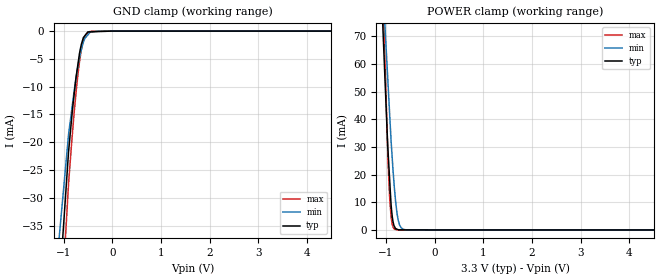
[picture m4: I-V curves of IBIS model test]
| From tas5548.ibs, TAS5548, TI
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|   test Model
[Model]   test
Model_type   Input
Vinl = 0.8
Vinh = 2
|   typ   min   max
|   (nom PVT)   (fast PVT)   (slow PVT)
|C_comp from frequency sweep method (F=50MHz)
|Average
|C_comp   1.354e-12   1.299e-12   1.358e-12
|C_comp from LC tank measurement(L=1nH)
|Average
|Resonant Frequency(Hz)   4.890e+09   4.950e+09   4.860e+09
C_comp   1.060e-12   1.035e-12   1.073e-12
| Where nom  PVT is Nominal Process, 3.3V, 27C
|   Fast PVT is Strong Process,  3.6V, 0C
|   Slow PVT is Weak Process,   3V, 125C
[Voltage Range]   3.3   3   3.6
|Ambient Temperature   27   125   0
|Junction Temperature
[Temperature Range]   27   125   0
[Power Clamp Reference]   3.3   3   3.6
[GND Clamp Reference]   0   0   0
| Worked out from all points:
|   GND clamp passes 1 mA (typ) near -0.58 V on its own axis
|   POWER clamp passes 1 mA (typ) near -0.82 V on its own axis
[GND Clamp]
|   Voltage   I(typ)   I(min)   I(max)
-3.3V     -1.788A    -1.552A    -1.885A
-1.541V   -104.9mA   -80.39mA   -124.7mA
-897.6mV  -21.73mA   -18.63mA   -27.52mA
-818.4mV  -14.27mA   -13.23mA   -18.46mA
-781.2mV  -11.3mA    -10.7mA    -14.55mA
-745.8mV  -8.478mA   -8.555mA   -11.3mA
-680.4mV  -4.492mA   -5.197mA   -6.037mA
-633.6mV  -2.361mA   -3.294mA   -3.31mA
-594mV    -1.214mA   -2.013mA   -1.73mA
-501.6mV  -157.3uA   -693uA     -238.7uA
-285mV    -88.9uA    -3.885uA   -18.49uA
6.6V      0A         0A         0A
[POWER Clamp]
|   Voltage   I(typ)   I(min)   I(max)
-3.3V     1.271A     947.8mA    1.891A
-1.063V   71.92mA    86.78mA    87.41mA
-1.04V    62.38mA    79.47mA    71.65mA
-957.6mV  27.91mA    52.23mA    23.83mA
-925.2mV  17.86mA    41.58mA    11.3mA
-884.4mV  6.686mA    28.92mA    3.276mA
-858mV    3.103mA    21.91mA    1.235mA
-817.2mV  915.8uA    12.92mA    226.5uA
-771mV    251.3uA    5.599mA    34.82uA
-723mV    45uA       1.841mA    5.304uA
-591mV    36.75uA    53.72uA    2.169uA
6.6V      0A         0A         0A
